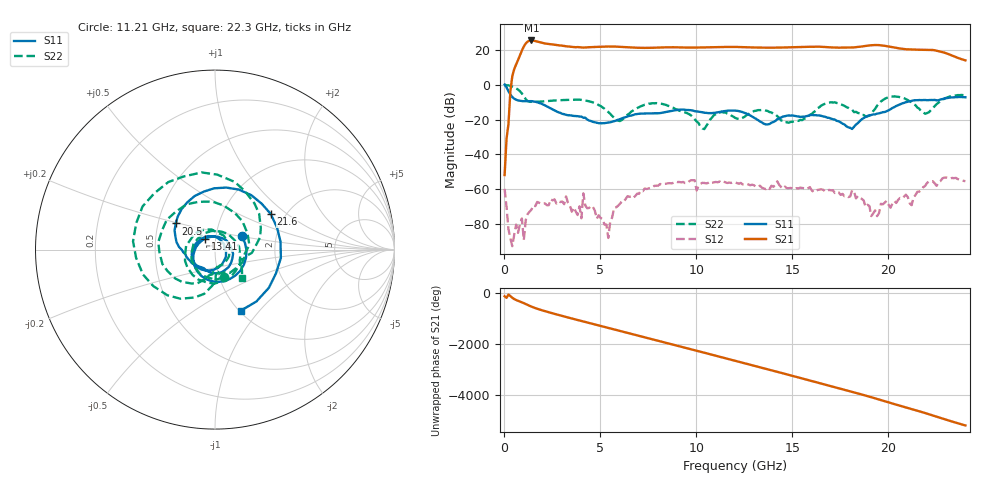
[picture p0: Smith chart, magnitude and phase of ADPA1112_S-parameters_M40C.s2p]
! Analog Devices Inc.
! Device:  ADPA1112
! Description: 15 W, GaN Power Amplifier
! Frequency:  1 GHz to 22 GHz
! Package:
! Conditions:	Vdd = 28.0 V
!		Idd = 600 mA
!		Temp = -40 C
! The board loss has been subtracted from S21 Magnitude. Reference for all other parameters are at the connectors.
! Misc:JB
! Note: Analog Devices supplies this data as a sample of measured data for this product.
! Your particular data for this product may vary.
! Analog Devices reserves the right to change this data at anytime
! Freq(GHz)	S11a(dB)	S11p(deg)	S21a(dB)	S21p(deg)	S12a(dB)	S12p(deg)	S22a(dB)	S22p(deg)
# GHz S  dB  R 50
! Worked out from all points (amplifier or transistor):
!   241 points, 10 MHz to 24 GHz, reference 50 ohm
!   highest |S21| = 25.6 dB at 1.41 GHz (marker M1)
!   |S21| within 3 dB of that: 1.037 GHz to 2.984 GHz (1.947 GHz wide, 96.9 % of centre)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
!   unconditionally stable (mu >= 1): 109 MHz to end of sweep
!   at 4.009 GHz: K = 241.01, MAG = 22.4 dB, |S12| = -76.7 dB
!   at 12.01 GHz: K = 24.24, MAG = 22.1 dB, |S12| = -56.0 dB
!   at 24 GHz: K = 34.44, MAG = 16.4 dB, |S12| = -55.4 dB
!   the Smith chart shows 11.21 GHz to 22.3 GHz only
!   S11 on the Smith chart (normalised r, x): 11.21 GHz: 1.34, +0.20; 13.41 GHz: 0.89, +0.11; 20.5 GHz: 0.62, +0.19; 21.6 GHz: 1.68, +0.77; 22.3 GHz: 1.02, -0.80
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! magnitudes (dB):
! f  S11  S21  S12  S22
! 10 MHz  0.2  -51.9  -59.8  0.2
! 209.9 MHz  -3.6  -22.5  -83.0  -0.2
! 409.9 MHz  -6.9  5.0  -92.8  -1.0
! 1.41 GHz  -9.3  25.6  -71.7  -9.7
! 3.209 GHz  -17.2  22.3  -64.1  -8.6
! 4.009 GHz  -18.2  21.7  -76.7  -8.6
! 4.109 GHz  -18.8  21.5  -62.4  -8.8
! 5.409 GHz  -21.6  22.1  -88.1  -15.5
! 6.408 GHz  -18.1  21.7  -64.1  -17.1
! 8.108 GHz  -16.2  21.6  -57.0  -10.7
! 10.41 GHz  -15.9  21.7  -56.4  -25.4
! 11.21 GHz  -15.5  21.8  -55.6  -15.9
! 12.01 GHz  -14.8  21.9  -56.0  -18.9
! 13.41 GHz  -21.6  21.5  -59.1  -14.4
! 16.01 GHz  -17.2  22.0  -60.7  -16.6
! 18.11 GHz  -25.3  21.6  -60.6  -14.3
! 19.11 GHz  -17.2  22.9  -75.5  -16.9
! 20.1 GHz  -14.0  22.0  -70.7  -6.8
! 20.5 GHz  -11.6  21.2  -66.1  -6.8
! 21.6 GHz  -8.7  20.3  -61.4  -13.7
! 22.3 GHz  -8.7  20.1  -55.4  -13.3
! 24 GHz  -7.1  14.2  -55.4  -5.8
